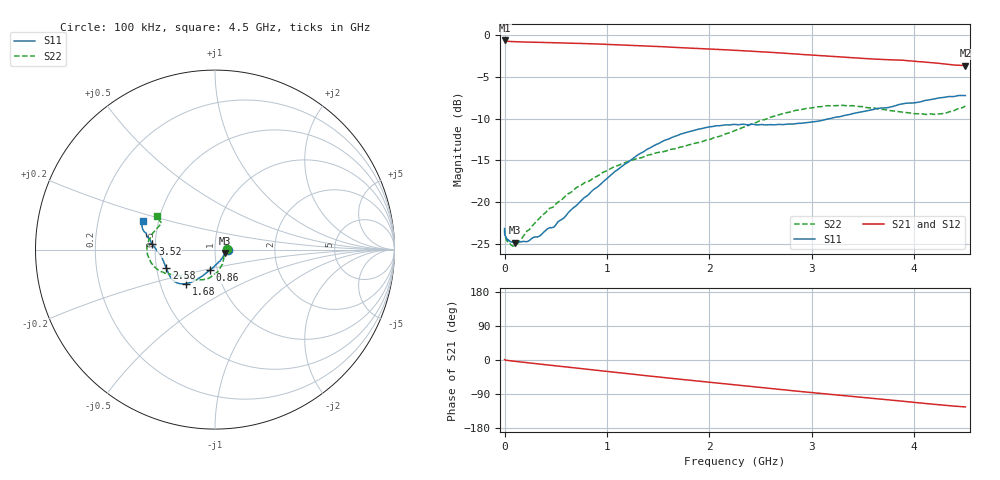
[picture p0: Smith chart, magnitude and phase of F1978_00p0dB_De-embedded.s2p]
! Integrated Device Technology
! Corporate Headquarters
! 6024 Silver Creek Valley Road
! San Jose, CA 95138  USA
! Phone:  1-408-284-8200
! Toll Free:  1-800-223-1366
! Webpage:  http://www.idt.com/
! Timing and RF Division
! 515 Groton Road, Suite 102
! Westford, MA 01886-6024
! Device:  F1978
! Description: 6-bit, 75 ohm, 0.5 dB Digital Step Attenuator
! Frequency:  5.0 MHz -  3.00 GHz
! Package:  4x4 mm QFN Plastic Package: 20 pin
! Ports:  2 RF, 11 DC
!  Pin  1  = D5 (16 dB)
!  Pin  2  = RF1  =  Port 1
!  Pin  3  = Serial Data In (DATA)
!  Pin  4  = Serial Clock (CLK)
!  Pin  5  = Serial Latch Enable (LE)
!  Pin  6  = VDD
!  Pin  7  = NC
!  Pin  8  = NC
!  Pin  9  = NC
!  Pin 10  = GND
!  Pin 11  = GND
!  Pin 12  = NC
!  Pin 13  = VMODE
!  Pin 14  = RF2  =  Port 2
!  Pin 15  = D4 (8 dB)
!  Pin 16  = D3 (4 dB)
!  Pin 17  = D2 (2 dB)
!  Pin 18  = NC
!  Pin 19  = D1 (1 dB)
!  Pin 20  = D0 (0.5 dB)
! State:  0
! Atten State:  0.0 dB
! Voltage:  +3.30 Volts
! Current:  0.593 mA
! Data:  The device was measured on a F1975 evaluation board which has
!  individual transmission lines to the RF pins.  Data was collected
!  using a calibrated network analyzer.  The evaluation board was
!  de-embedded using Automatic Fixture Removal (AFR).
!  The reference plane is the edge of the package pin.
! Misc:
!  Action Tracker AT0416
! Date Measured:  2018-02-08
! Date:  2018-03-26  MJV
! Note:
!  Integrated Device Technology supplies this data as a sample of measured
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# GHz S dB R 75
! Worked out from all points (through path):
!   291 points, 100 kHz to 4.5 GHz, reference 75 ohm
!   highest |S21| = -0.66 dB at 100 kHz (marker M1); lowest = -3.7 dB at 4.5 GHz (marker M2)
!   group delay of S21, straight-line fit = 77.7 ps
!   lowest |S11| = -24.8 dB at 100 MHz (marker M3), VSWR 1.12, Z = 83.5 - j3.22 ohm
!   |S11| at or under -10 dB: start of sweep to 3.179 GHz
!   |S22| runs from -25.2 to -8.4 dB; largest |S21 - S12| = 0.00027
!   S11 on the Smith chart (normalised r, x): 100 kHz: 1.15, +0.00; 860 MHz: 0.92, -0.21; 1.68 GHz: 0.68, -0.27; 2.58 GHz: 0.56, -0.13; 3.52 GHz: 0.48, +0.03; 4.5 GHz: 0.41, +0.16
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0.0001  -23.14 0.2  -0.66 1.2  -0.67 1.2  -23.26 0.8
0.0005  -23.56 -1.3  -0.69 1.1  -0.69 1.0  -23.60 -0.3
0.002  -23.86 -1.2  -0.71 0.8  -0.71 0.8  -23.95 -0.4
0.02  -24.34 -5.9  -0.75 -0.9  -0.75 -0.9  -24.59 -6.5
0.1  -24.82 -19.6  -0.81 -3.4  -0.81 -3.4  -25.20 -22.8
0.22  -24.71 -38.3  -0.85 -7.1  -0.85 -7.1  -23.42 -43.3
0.44  -23.04 -66.4  -0.92 -13.6  -0.92 -13.6  -20.71 -63.2
0.48  -22.98 -72.0  -0.94 -14.8  -0.93 -14.8  -20.52 -67.0
0.76  -19.66 -97.7  -1.03 -23.1  -1.03 -23.1  -17.85 -85.5
0.86  -18.57 -103.8  -1.07 -26.1  -1.07 -26.1  -17.18 -91.8
1.08  -16.30 -113.5  -1.16 -32.6  -1.16 -32.6  -15.68 -102.7
1.52  -12.88 -126.4  -1.40 -45.3  -1.40 -45.3  -14.02 -122.1
1.68  -12.06 -130.6  -1.50 -49.8  -1.50 -49.8  -13.57 -129.1
1.96  -11.08 -138.1  -1.67 -57.6  -1.67 -57.6  -12.61 -140.0
2.26  -10.71 -147.3  -1.85 -65.9  -1.85 -65.9  -11.38 -148.7
2.58  -10.73 -159.0  -2.07 -74.7  -2.07 -74.7  -9.92 -157.0
3.02  -10.39 -173.2  -2.42 -86.5  -2.42 -86.5  -8.68 -170.8
3.3  -9.69 179.8  -2.67 -93.8  -2.66 -93.8  -8.42 178.3
3.52  -9.12 175.0  -2.82 -99.3  -2.82 -99.3  -8.63 170.9
3.76  -8.64 170.7  -2.97 -105.2  -2.97 -105.2  -9.04 163.6
4.22  -7.57 164.2  -3.36 -117.6  -3.36 -117.6  -9.50 153.4
4.5  -7.25 158.4  -3.66 -123.9  -3.66 -123.9  -8.50 149.7
